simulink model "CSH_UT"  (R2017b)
settings: Solver=FixedStepDiscrete  StartTime=0.0  StopTime=10.0  FixedStep=0.01  RelTol=1e-3  EnableMultiTasking=on
undefined symbols (not defined in the file): ASWTYPE_FALSE, CbCSH_CANCrashFltDetEnable_flg, CcCSH_CshDutyNormalHi_pct, CcCSH_CshDutyNormalLo_pct, CcCSH_CshFltDutyHiThrd_pct, CcCSH_CshFltDutyLoThrd_pct, CcCSH_CshFrqNormalHi_ms, CcCSH_CshFrqNormalLo_ms, CcCSH_DutyAbnormalDetEnable_flg, CcCSH_FrqAbnormalDetEnable_flg, CcCSH_HWCshFltDetEnable_flg, CcCSH_Kl15WkUpDelay_ms, CSH_CONST10_NUMB, CSH_CONST11_NUMB, CSH_CONST16_NUMB, CSH_CONST17_NUMB, CSH_CONST18_NUMB, CSH_CONST19_NUMB, CSH_CONST1_NUMB, CSH_CONST24_NUMB, CSH_CONST25_NUMB, CSH_CONST26_NUMB, CSH_CONST27_NUMB, CSH_CONST2_NUMB, CSH_CONST3_NUMB, CSH_CONST4_NUMB, CSH_CONST5_NUMB, CSH_CONST6_NUMB, CSH_CONST7_NUMB, CSH_CONST8_NUMB, CSH_CONST9_NUMB, CSH_RUNTIME_MS
libraries: AIWAYS_Powertrain_BMS_lib x11

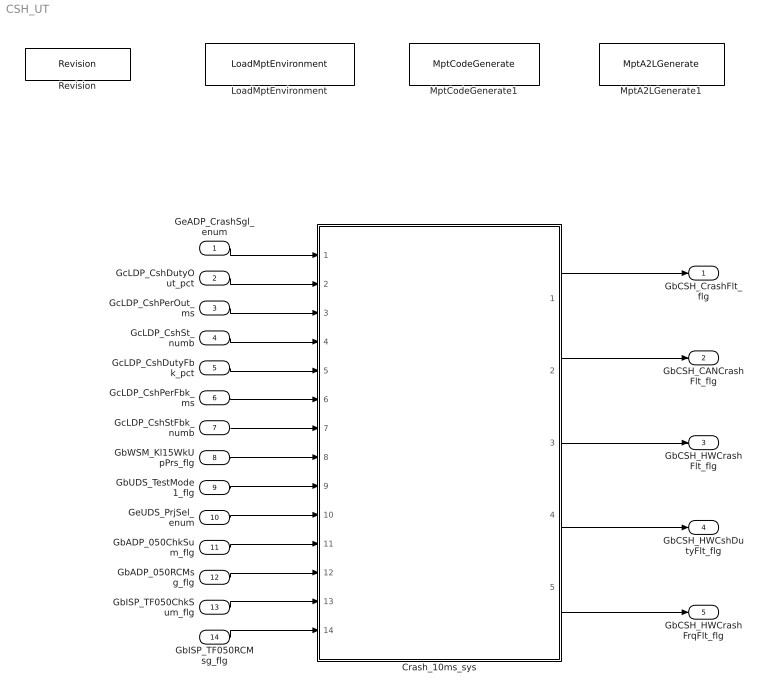
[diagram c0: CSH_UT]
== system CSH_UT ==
  GeADP_CrashSgl_enum : Inport
  GcLDP_CshDutyOut_pct : Inport  Port=2
  GcLDP_CshPerOut_ms : Inport  Port=3
  GcLDP_CshSt_numb : Inport  Port=4
  GcLDP_CshDutyFbk_pct : Inport  Port=5
  GcLDP_CshPerFbk_ms : Inport  Port=6
  GcLDP_CshStFbk_numb : Inport  Port=7
  GbWSM_Kl15WkUpPrs_flg : Inport  Port=8
  GbUDS_TestMode1_flg : Inport  Port=9
  GeUDS_PrjSel_enum : Inport  Port=10
  GbADP_050ChkSum_flg : Inport  Port=11
  GbADP_050RCMsg_flg : Inport  Port=12
  GbISP_TF050ChkSum_flg : Inport  Port=13
  GbISP_TF050RCMsg_flg : Inport  Port=14
  Crash_10ms_sys : Subsystem
  LoadMptEnvironment : AIWAYS_Powertrain_BMS_lib/Config/LoadMptEnvironment  ProjectName=Comm  SuppierID=NewPlatformUAES
  MptA2LGenerate1 : AIWAYS_Powertrain_BMS_lib/Config/MptA2LGenerate  SystemSampleTime=-1
  MptCodeGenerate1 : AIWAYS_Powertrain_BMS_lib/Config/MptCodeGenerate  SystemSampleTime=-1
  Revision : AIWAYS_Powertrain_BMS_lib/Config/Revision  curVersion='M102C102'  newVersion='M102C102'
  GbCSH_CrashFlt_flg : Outport
  GbCSH_CANCrashFlt_flg : Outport  Port=2
  GbCSH_HWCrashFlt_flg : Outport  Port=3
  GbCSH_HWCshDutyFlt_flg : Outport  Port=4
  GbCSH_HWCrashFrqFlt_flg : Outport  Port=5
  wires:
  GcLDP_CshPerOut_ms/1 -> Crash_10ms_sys/3(GcLDP_CshPerOut_ms)
  GcLDP_CshStFbk_numb/1 -> Crash_10ms_sys/7(GcLDP_CshStFbk_numb)
  GbWSM_Kl15WkUpPrs_flg/1 -> Crash_10ms_sys/8(GbWSM_Kl15WkUpPrs_flg)
  Crash_10ms_sys/5(GbCSH_HWCrashFrqFlt_flg) -> GbCSH_HWCrashFrqFlt_flg/1
  GcLDP_CshPerFbk_ms/1 -> Crash_10ms_sys/6(GcLDP_CshPerFbk_ms)
  Crash_10ms_sys/3(GbCSH_HWCrashFlt_flg) -> GbCSH_HWCrashFlt_flg/1
  GbUDS_TestMode1_flg/1 -> Crash_10ms_sys/9(GbUDS_TestMode1_flg)
  Crash_10ms_sys/1(GbCSH_CrashFlt_flg) -> GbCSH_CrashFlt_flg/1
  GeADP_CrashSgl_enum/1 -> Crash_10ms_sys/1(GeADP_CrashSgl_enum)
  GcLDP_CshDutyFbk_pct/1 -> Crash_10ms_sys/5(GcLDP_CshDutyFbk_pct)
  GeUDS_PrjSel_enum/1 -> Crash_10ms_sys/10(GeUDS_PrjSel_enum)
  Crash_10ms_sys/2(GbCSH_CANCrashFlt_flg) -> GbCSH_CANCrashFlt_flg/1
  GbISP_TF050RCMsg_flg/1 -> Crash_10ms_sys/14(GbISP_TF050RCMsg_flg)
  GcLDP_CshSt_numb/1 -> Crash_10ms_sys/4(GcLDP_CshSt_numb)
  GbADP_050ChkSum_flg/1 -> Crash_10ms_sys/11(GbADP_050ChkSum_flg)
  GcLDP_CshDutyOut_pct/1 -> Crash_10ms_sys/2(GcLDP_CshDutyOut_pct)
  Crash_10ms_sys/4(GbCSH_HWCshDutyFlt_flg) -> GbCSH_HWCshDutyFlt_flg/1
  GbADP_050RCMsg_flg/1 -> Crash_10ms_sys/12(GbADP_050RCMsg_flg)
  GbISP_TF050ChkSum_flg/1 -> Crash_10ms_sys/13(GbISP_TF050ChkSum_flg)

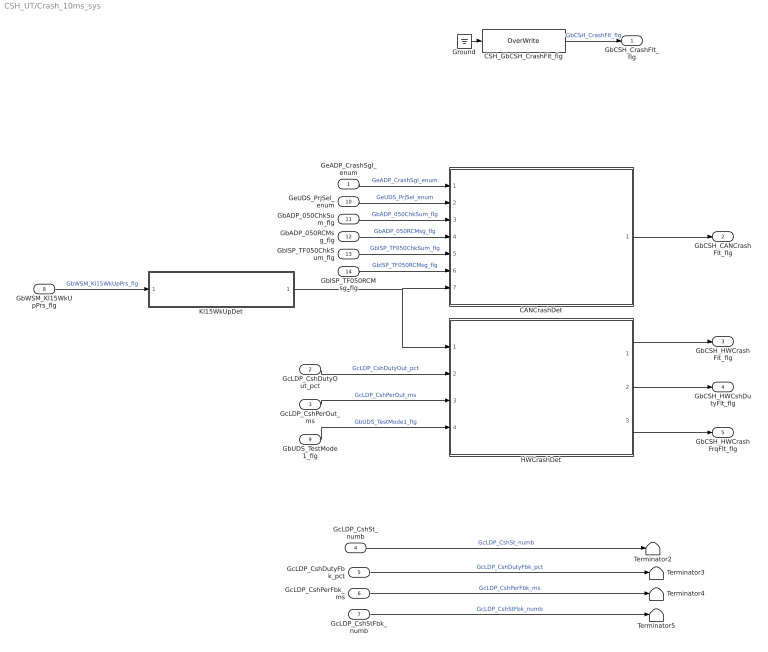
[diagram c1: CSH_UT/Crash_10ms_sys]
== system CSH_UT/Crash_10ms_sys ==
  GeADP_CrashSgl_enum : Inport
  GcLDP_CshDutyOut_pct : Inport  Port=2
  GcLDP_CshPerOut_ms : Inport  Port=3
  GcLDP_CshSt_numb : Inport  Port=4
  GcLDP_CshDutyFbk_pct : Inport  Port=5
  GcLDP_CshPerFbk_ms : Inport  Port=6
  GcLDP_CshStFbk_numb : Inport  Port=7
  GbWSM_Kl15WkUpPrs_flg : Inport  Port=8
  GbUDS_TestMode1_flg : Inport  Port=9
  GeUDS_PrjSel_enum : Inport  Port=10
  GbADP_050ChkSum_flg : Inport  Port=11
  GbADP_050RCMsg_flg : Inport  Port=12
  GbISP_TF050ChkSum_flg : Inport  Port=13
  GbISP_TF050RCMsg_flg : Inport  Port=14
  CANCrashDet : Subsystem
  CSH_GbCSH_CrashFlt_flg : AIWAYS_Powertrain_BMS_lib/Signals/OverWrite  OverWrite_Value=CbCSH_CrashFltOvr_flg  OverWrite_flag=CbCSH_CrashFltOvrSwt_flg
  Ground : Ground
  HWCrashDet : Subsystem
  Kl15WkUpDet : Subsystem
  Terminator{2..5} (4 alike) : Terminator
  GbCSH_CrashFlt_flg : Outport
  GbCSH_CANCrashFlt_flg : Outport  Port=2
  GbCSH_HWCrashFlt_flg : Outport  Port=3
  GbCSH_HWCshDutyFlt_flg : Outport  Port=4
  GbCSH_HWCrashFrqFlt_flg : Outport  Port=5
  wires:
  GeADP_CrashSgl_enum/1 -> CANCrashDet/1(GeADP_CrashSgl_enum)  "GeADP_CrashSgl_enum"
  CSH_GbCSH_CrashFlt_flg/1 -> GbCSH_CrashFlt_flg/1  "GbCSH_CrashFlt_flg"
  GcLDP_CshDutyOut_pct/1 -> HWCrashDet/2(GcLDP_CshDutyOut_pct)  "GcLDP_CshDutyOut_pct"
  GcLDP_CshPerOut_ms/1 -> HWCrashDet/3(GcLDP_CshPerOut_ms)  "GcLDP_CshPerOut_ms"
  GcLDP_CshSt_numb/1 -> Terminator2/1  "GcLDP_CshSt_numb"
  GcLDP_CshDutyFbk_pct/1 -> Terminator3/1  "GcLDP_CshDutyFbk_pct"
  GcLDP_CshPerFbk_ms/1 -> Terminator4/1  "GcLDP_CshPerFbk_ms"
  GcLDP_CshStFbk_numb/1 -> Terminator5/1  "GcLDP_CshStFbk_numb"
  Ground/1 -> CSH_GbCSH_CrashFlt_flg/1
  GbWSM_Kl15WkUpPrs_flg/1 -> Kl15WkUpDet/1(GbWSM_Kl15WkUpPrs_flg)  "GbWSM_Kl15WkUpPrs_flg"
  Kl15WkUpDet/1(LbCSH_Kl15WkUpPrs_flg) -> HWCrashDet/1(LbCSH_Kl15WkUpPrs_flg), CANCrashDet/7(LbCSH_Kl15WkUpPrs_flg)
  GbUDS_TestMode1_flg/1 -> HWCrashDet/4(GbUDS_TestMode1_flg)  "GbUDS_TestMode1_flg"
  GeUDS_PrjSel_enum/1 -> CANCrashDet/2(GeUDS_PrjSel_enum)  "GeUDS_PrjSel_enum"
  HWCrashDet/1(GbCSH_HWCrashFlt_flg) -> GbCSH_HWCrashFlt_flg/1
  HWCrashDet/2(GbCSH_HWCshDutyFlt_flg) -> GbCSH_HWCshDutyFlt_flg/1
  HWCrashDet/3(GbCSH_HWCrashFrqFlt_flg) -> GbCSH_HWCrashFrqFlt_flg/1
  GbADP_050ChkSum_flg/1 -> CANCrashDet/3(GbADP_050ChkSum_flg)  "GbADP_050ChkSum_flg"
  GbADP_050RCMsg_flg/1 -> CANCrashDet/4(GbADP_050RCMsg_flg)  "GbADP_050RCMsg_flg"
  GbISP_TF050ChkSum_flg/1 -> CANCrashDet/5(GbISP_TF050ChkSum_flg)  "GbISP_TF050ChkSum_flg"
  GbISP_TF050RCMsg_flg/1 -> CANCrashDet/6(GbISP_TF050RCMsg_flg)  "GbISP_TF050RCMsg_flg"
  CANCrashDet/1(GbCSH_CANCrashFlt_flg) -> GbCSH_CANCrashFlt_flg/1

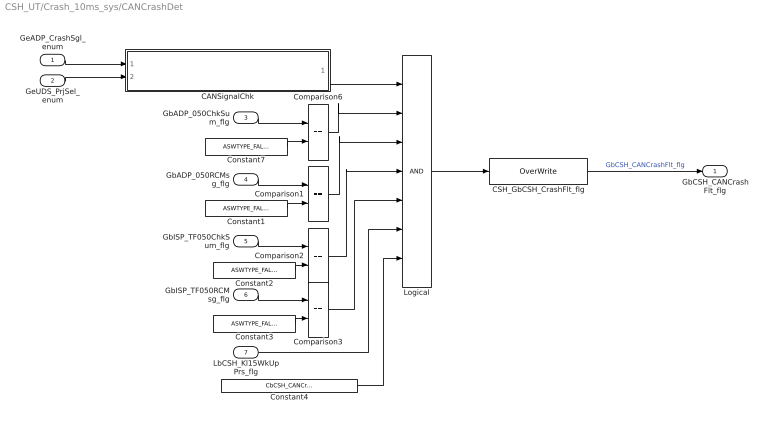
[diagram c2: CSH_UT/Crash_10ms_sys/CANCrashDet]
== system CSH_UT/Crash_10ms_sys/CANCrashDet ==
  GeADP_CrashSgl_enum : Inport
  GeUDS_PrjSel_enum : Inport  Port=2
  GbADP_050ChkSum_flg : Inport  Port=3
  GbADP_050RCMsg_flg : Inport  Port=4
  GbISP_TF050ChkSum_flg : Inport  Port=5
  GbISP_TF050RCMsg_flg : Inport  Port=6
  LbCSH_Kl15WkUpPrs_flg : Inport  Port=7
  CANSignalChk : Subsystem
  CSH_GbCSH_CrashFlt_flg : AIWAYS_Powertrain_BMS_lib/Signals/OverWrite  OverWrite_Value=CbCSH_CANCrashFltOvr_flg  OverWrite_flag=CbCSH_CANCrashFltOvrSwt_flg
  Comparison{1..3,6} (4 alike) : RelationalOperator  Operator===  OutDataTypeStr=boolean
  Constant{1..3,7} (4 alike) : Constant  Value=ASWTYPE_FALSE
  Constant4 : Constant  Value=CbCSH_CANCrashFltDetEnable_flg
  Logical : Logic  Inputs=7  OutDataTypeStr=boolean
  GbCSH_CANCrashFlt_flg : Outport
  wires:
  LbCSH_Kl15WkUpPrs_flg/1 -> Logical/6
  GeADP_CrashSgl_enum/1 -> CANSignalChk/1(GeADP_CrashSgl_enum)
  GeUDS_PrjSel_enum/1 -> CANSignalChk/2(GeUDS_PrjSel_enum)
  Constant7/1 -> Comparison6/2
  GbADP_050ChkSum_flg/1 -> Comparison6/1
  Constant1/1 -> Comparison1/2
  GbADP_050RCMsg_flg/1 -> Comparison1/1
  CANSignalChk/1(LbCSH_CANCrashState_flg) -> Logical/1
  Comparison6/1 -> Logical/2
  Comparison1/1 -> Logical/3
  GbISP_TF050ChkSum_flg/1 -> Comparison2/1
  Constant2/1 -> Comparison2/2
  Comparison2/1 -> Logical/4
  GbISP_TF050RCMsg_flg/1 -> Comparison3/1
  Constant3/1 -> Comparison3/2
  Comparison3/1 -> Logical/5
  Logical/1 -> CSH_GbCSH_CrashFlt_flg/1
  CSH_GbCSH_CrashFlt_flg/1 -> GbCSH_CANCrashFlt_flg/1  "GbCSH_CANCrashFlt_flg"
  Constant4/1 -> Logical/7

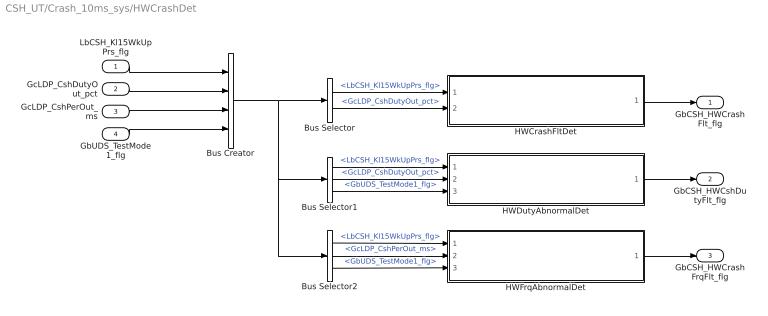
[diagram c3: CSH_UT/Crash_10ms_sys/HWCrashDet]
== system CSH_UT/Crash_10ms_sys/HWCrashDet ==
  LbCSH_Kl15WkUpPrs_flg : Inport
  GcLDP_CshDutyOut_pct : Inport  Port=2
  GcLDP_CshPerOut_ms : Inport  Port=3
  GbUDS_TestMode1_flg : Inport  Port=4
  Bus Creator : BusCreator  Inputs=4
  Bus Selector : BusSelector  OutputSignals=LbCSH_Kl15WkUpPrs_flg,GcLDP_CshDutyOut_pct
  Bus Selector1 : BusSelector  OutputSignals=LbCSH_Kl15WkUpPrs_flg,GcLDP_CshDutyOut_pct,GbUDS_TestMode1_flg
  Bus Selector2 : BusSelector  OutputSignals=LbCSH_Kl15WkUpPrs_flg,GcLDP_CshPerOut_ms,GbUDS_TestMode1_flg
  HWCrashFltDet : Subsystem
  HWDutyAbnormalDet : Subsystem
  HWFrqAbnormalDet : Subsystem
  GbCSH_HWCrashFlt_flg : Outport
  GbCSH_HWCshDutyFlt_flg : Outport  Port=2
  GbCSH_HWCrashFrqFlt_flg : Outport  Port=3
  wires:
  LbCSH_Kl15WkUpPrs_flg/1 -> Bus Creator/1
  GcLDP_CshDutyOut_pct/1 -> Bus Creator/2
  GcLDP_CshPerOut_ms/1 -> Bus Creator/3
  Bus Creator/1 -> Bus Selector2/1, Bus Selector1/1, Bus Selector/1
  Bus Selector/1 -> HWCrashFltDet/1(LbCSH_Kl15WkUpPrs_flg)  "<LbCSH_Kl15WkUpPrs_flg>"
  Bus Selector/2 -> HWCrashFltDet/2(GcLDP_CshDutyOut_pct)  "<GcLDP_CshDutyOut_pct>"
  GbUDS_TestMode1_flg/1 -> Bus Creator/4
  HWCrashFltDet/1(GbCSH_HWCrashFlt_flg) -> GbCSH_HWCrashFlt_flg/1
  Bus Selector1/1 -> HWDutyAbnormalDet/1(LbCSH_Kl15WkUpPrs_flg)  "<LbCSH_Kl15WkUpPrs_flg>"
  Bus Selector1/2 -> HWDutyAbnormalDet/2(GcLDP_CshDutyOut_pct)  "<GcLDP_CshDutyOut_pct>"
  Bus Selector1/3 -> HWDutyAbnormalDet/3(GbUDS_TestMode1_flg)  "<GbUDS_TestMode1_flg>"
  Bus Selector2/1 -> HWFrqAbnormalDet/1(LbCSH_Kl15WkUpPrs_flg)  "<LbCSH_Kl15WkUpPrs_flg>"
  Bus Selector2/2 -> HWFrqAbnormalDet/2(GcLDP_CshPerOut_ms)  "<GcLDP_CshPerOut_ms>"
  Bus Selector2/3 -> HWFrqAbnormalDet/3(GbUDS_TestMode1_flg)  "<GbUDS_TestMode1_flg>"
  HWDutyAbnormalDet/1(GbCSH_HWCshDutyFlt_flg) -> GbCSH_HWCshDutyFlt_flg/1
  HWFrqAbnormalDet/1(GbCSH_HWCrashFrqFlt_flg) -> GbCSH_HWCrashFrqFlt_flg/1

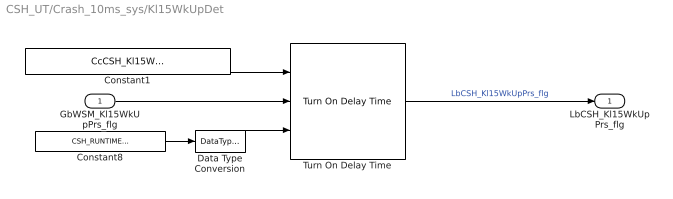
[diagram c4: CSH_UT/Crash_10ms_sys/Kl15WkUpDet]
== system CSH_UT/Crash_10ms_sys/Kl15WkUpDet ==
  GbWSM_Kl15WkUpPrs_flg : Inport
  Constant1 : Constant  Value=CcCSH_Kl15WkUpDelay_ms
  Constant8 : Constant  Value=CSH_RUNTIME_MS
  Data Type Conversion : DataTypeConversion
  Turn On Delay Time : AIWAYS_Powertrain_BMS_lib/Delay Blocks/Turn On Delay Time
  LbCSH_Kl15WkUpPrs_flg : Outport
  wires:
  GbWSM_Kl15WkUpPrs_flg/1 -> Turn On Delay Time/2
  Constant8/1 -> Data Type Conversion/1
  Constant1/1 -> Turn On Delay Time/1
  Turn On Delay Time/1 -> LbCSH_Kl15WkUpPrs_flg/1  "LbCSH_Kl15WkUpPrs_flg"
  Data Type Conversion/1 -> Turn On Delay Time/3

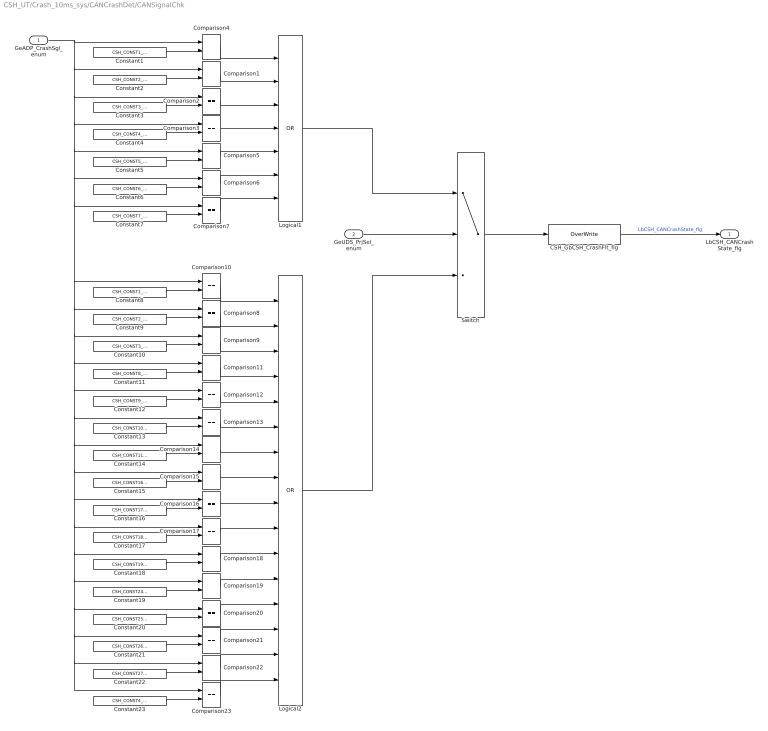
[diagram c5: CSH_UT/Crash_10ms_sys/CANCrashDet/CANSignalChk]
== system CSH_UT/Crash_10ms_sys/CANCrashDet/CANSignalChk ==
  GeADP_CrashSgl_enum : Inport
  GeUDS_PrjSel_enum : Inport  Port=2
  CSH_GbCSH_CrashFlt_flg : AIWAYS_Powertrain_BMS_lib/Signals/OverWrite  OverWrite_Value=CbCSH_CANCrashStateOvr_flg  OverWrite_flag=CbCSH_CANCrashStateOvrSwt_flg
  Comparison{1..23} (23 alike) : RelationalOperator  Operator===  OutDataTypeStr=boolean
  Constant1 : Constant  Value=CSH_CONST1_NUMB
  Constant10 : Constant  Value=CSH_CONST3_NUMB
  Constant11 : Constant  Value=CSH_CONST8_NUMB
  Constant12 : Constant  Value=CSH_CONST9_NUMB
  Constant13 : Constant  Value=CSH_CONST10_NUMB
  Constant14 : Constant  Value=CSH_CONST11_NUMB
  Constant15 : Constant  Value=CSH_CONST16_NUMB
  Constant16 : Constant  Value=CSH_CONST17_NUMB
  Constant17 : Constant  Value=CSH_CONST18_NUMB
  Constant18 : Constant  Value=CSH_CONST19_NUMB
  Constant19 : Constant  Value=CSH_CONST24_NUMB
  Constant2 : Constant  Value=CSH_CONST2_NUMB
  Constant20 : Constant  Value=CSH_CONST25_NUMB
  Constant21 : Constant  Value=CSH_CONST26_NUMB
  Constant22 : Constant  Value=CSH_CONST27_NUMB
  Constant23 : Constant  Value=CSH_CONST4_NUMB
  Constant3 : Constant  Value=CSH_CONST3_NUMB
  Constant4 : Constant  Value=CSH_CONST4_NUMB
  Constant5 : Constant  Value=CSH_CONST5_NUMB
  Constant6 : Constant  Value=CSH_CONST6_NUMB
  Constant7 : Constant  Value=CSH_CONST7_NUMB
  Constant8 : Constant  Value=CSH_CONST1_NUMB
  Constant9 : Constant  Value=CSH_CONST2_NUMB
  Logical1 : Logic  Operator=OR  Inputs=7  OutDataTypeStr=boolean
  Logical2 : Logic  Operator=OR  Inputs=16  OutDataTypeStr=boolean
  Switch : Switch  Criteria=u2 ~= 0  Threshold=1  RndMeth=Zero
  LbCSH_CANCrashState_flg : Outport
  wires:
  Constant1/1 -> Comparison4/2
  Constant2/1 -> Comparison1/2
  Constant3/1 -> Comparison2/2
  Constant4/1 -> Comparison3/2
  Constant5/1 -> Comparison5/2
  Constant6/1 -> Comparison6/2
  Constant7/1 -> Comparison7/2
  Comparison4/1 -> Logical1/1
  Comparison1/1 -> Logical1/2
  Comparison2/1 -> Logical1/3
  Comparison3/1 -> Logical1/4
  Comparison5/1 -> Logical1/5
  Comparison6/1 -> Logical1/6
  Comparison7/1 -> Logical1/7
  GeADP_CrashSgl_enum/1 -> Comparison2/1, Comparison3/1, Comparison5/1, Comparison6/1, Comparison7/1, Comparison9/1, Comparison14/1, Comparison15/1, Comparison16/1, Comparison17/1, Comparison18/1, Comparison19/1, Comparison20/1, Comparison21/1, Comparison23/1, Comparison22/1, Comparison13/1, Comparison12/1, Comparison11/1, Comparison8/1, Comparison10/1, Comparison1/1, Comparison4/1
  Constant9/1 -> Comparison8/2
  Constant8/1 -> Comparison10/2
  Constant10/1 -> Comparison9/2
  Constant11/1 -> Comparison11/2
  Constant12/1 -> Comparison12/2
  Constant13/1 -> Comparison13/2
  Constant14/1 -> Comparison14/2
  Constant18/1 -> Comparison18/2
  Constant17/1 -> Comparison17/2
  Constant16/1 -> Comparison16/2
  Constant15/1 -> Comparison15/2
  Constant19/1 -> Comparison19/2
  Constant20/1 -> Comparison20/2
  Constant21/1 -> Comparison21/2
  Constant22/1 -> Comparison22/2
  Comparison10/1 -> Logical2/1
  Comparison8/1 -> Logical2/2
  Comparison9/1 -> Logical2/3
  Comparison11/1 -> Logical2/4
  Comparison12/1 -> Logical2/5
  Comparison13/1 -> Logical2/6
  Comparison14/1 -> Logical2/7
  Comparison15/1 -> Logical2/8
  Comparison16/1 -> Logical2/9
  Comparison17/1 -> Logical2/10
  Comparison18/1 -> Logical2/11
  Comparison19/1 -> Logical2/12
  Comparison20/1 -> Logical2/13
  Comparison21/1 -> Logical2/14
  Comparison22/1 -> Logical2/15
  Logical1/1 -> Switch/1
  GeUDS_PrjSel_enum/1 -> Switch/2
  Logical2/1 -> Switch/3
  Switch/1 -> CSH_GbCSH_CrashFlt_flg/1
  CSH_GbCSH_CrashFlt_flg/1 -> LbCSH_CANCrashState_flg/1  "LbCSH_CANCrashState_flg"
  Constant23/1 -> Comparison23/2
  Comparison23/1 -> Logical2/16

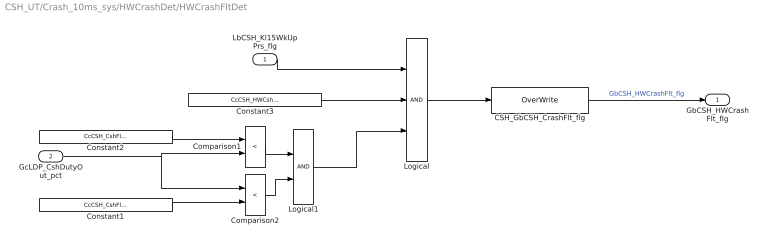
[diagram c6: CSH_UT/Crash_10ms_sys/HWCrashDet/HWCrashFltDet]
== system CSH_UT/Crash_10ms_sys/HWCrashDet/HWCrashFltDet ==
  LbCSH_Kl15WkUpPrs_flg : Inport
  GcLDP_CshDutyOut_pct : Inport  Port=2
  CSH_GbCSH_CrashFlt_flg : AIWAYS_Powertrain_BMS_lib/Signals/OverWrite  OverWrite_Value=CbCSH_HWCrashFltOvr_flg  OverWrite_flag=CbCSH_HWCrashFltOvrSwt_flg
  Comparison1 : RelationalOperator  Operator=<  OutDataTypeStr=boolean
  Comparison2 : RelationalOperator  Operator=<  OutDataTypeStr=boolean
  Constant1 : Constant  Value=CcCSH_CshFltDutyHiThrd_pct
  Constant2 : Constant  Value=CcCSH_CshFltDutyLoThrd_pct
  Constant3 : Constant  Value=CcCSH_HWCshFltDetEnable_flg
  Logical : Logic  Inputs=3  OutDataTypeStr=boolean
  Logical1 : Logic  OutDataTypeStr=boolean
  GbCSH_HWCrashFlt_flg : Outport
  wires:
  Constant1/1 -> Comparison2/2
  GcLDP_CshDutyOut_pct/1 -> Comparison2/1, Comparison1/2
  Constant2/1 -> Comparison1/1
  Comparison1/1 -> Logical1/1
  Comparison2/1 -> Logical1/2
  LbCSH_Kl15WkUpPrs_flg/1 -> Logical/1
  Constant3/1 -> Logical/2
  Logical1/1 -> Logical/3
  Logical/1 -> CSH_GbCSH_CrashFlt_flg/1
  CSH_GbCSH_CrashFlt_flg/1 -> GbCSH_HWCrashFlt_flg/1  "GbCSH_HWCrashFlt_flg"

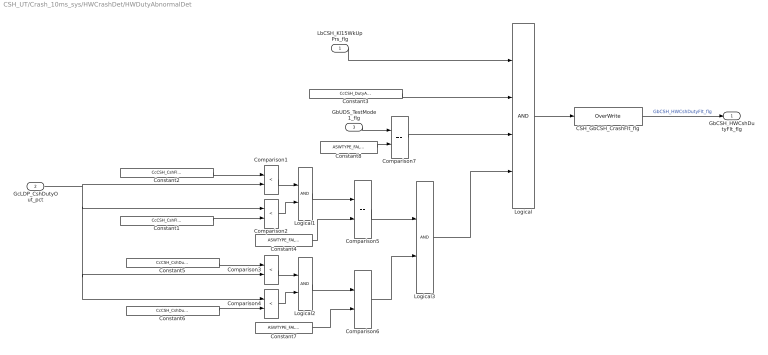
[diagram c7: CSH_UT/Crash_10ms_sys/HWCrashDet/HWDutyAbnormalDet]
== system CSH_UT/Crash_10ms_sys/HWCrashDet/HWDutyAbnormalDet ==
  LbCSH_Kl15WkUpPrs_flg : Inport
  GcLDP_CshDutyOut_pct : Inport  Port=2
  GbUDS_TestMode1_flg : Inport  Port=3
  CSH_GbCSH_CrashFlt_flg : AIWAYS_Powertrain_BMS_lib/Signals/OverWrite  OverWrite_Value=CbCSH_HWCshDutyFltOvr_flg  OverWrite_flag=CbCSH_HWCshDutyFltOvrSwt_flg
  Comparison{1..4} (4 alike) : RelationalOperator  Operator=<  OutDataTypeStr=boolean
  Comparison5 : RelationalOperator  Operator===  OutDataTypeStr=boolean
  Comparison6 : RelationalOperator  Operator===  OutDataTypeStr=boolean
  Comparison7 : RelationalOperator  Operator===  OutDataTypeStr=boolean
  Constant1 : Constant  Value=CcCSH_CshFltDutyHiThrd_pct
  Constant2 : Constant  Value=CcCSH_CshFltDutyLoThrd_pct
  Constant3 : Constant  Value=CcCSH_DutyAbnormalDetEnable_flg
  Constant4 : Constant  Value=ASWTYPE_FALSE
  Constant5 : Constant  Value=CcCSH_CshDutyNormalLo_pct
  Constant6 : Constant  Value=CcCSH_CshDutyNormalHi_pct
  Constant7 : Constant  Value=ASWTYPE_FALSE
  Constant8 : Constant  Value=ASWTYPE_FALSE
  Logical : Logic  Inputs=4  OutDataTypeStr=boolean
  Logical1 : Logic  OutDataTypeStr=boolean
  Logical2 : Logic  OutDataTypeStr=boolean
  Logical3 : Logic  OutDataTypeStr=boolean
  GbCSH_HWCshDutyFlt_flg : Outport
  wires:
  CSH_GbCSH_CrashFlt_flg/1 -> GbCSH_HWCshDutyFlt_flg/1  "GbCSH_HWCshDutyFlt_flg"
  Logical/1 -> CSH_GbCSH_CrashFlt_flg/1
  Logical1/1 -> Comparison5/1
  Constant3/1 -> Logical/2
  LbCSH_Kl15WkUpPrs_flg/1 -> Logical/1
  Comparison2/1 -> Logical1/2
  Comparison1/1 -> Logical1/1
  Constant2/1 -> Comparison1/1
  Constant1/1 -> Comparison2/2
  Constant5/1 -> Comparison3/1
  GcLDP_CshDutyOut_pct/1 -> Comparison1/2, Comparison3/2, Comparison4/1, Comparison2/1
  Constant6/1 -> Comparison4/2
  Comparison3/1 -> Logical2/1
  Comparison4/1 -> Logical2/2
  Constant4/1 -> Comparison5/2
  Logical2/1 -> Comparison6/1
  Constant7/1 -> Comparison6/2
  GbUDS_TestMode1_flg/1 -> Comparison7/1
  Constant8/1 -> Comparison7/2
  Comparison5/1 -> Logical3/1
  Comparison6/1 -> Logical3/2
  Comparison7/1 -> Logical/3
  Logical3/1 -> Logical/4

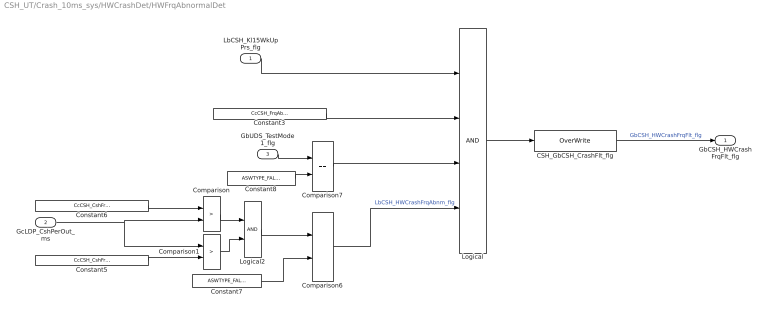
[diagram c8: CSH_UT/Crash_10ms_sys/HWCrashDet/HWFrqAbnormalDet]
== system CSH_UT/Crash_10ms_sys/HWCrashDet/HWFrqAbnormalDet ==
  LbCSH_Kl15WkUpPrs_flg : Inport
  GcLDP_CshPerOut_ms : Inport  Port=2
  GbUDS_TestMode1_flg : Inport  Port=3
  CSH_GbCSH_CrashFlt_flg : AIWAYS_Powertrain_BMS_lib/Signals/OverWrite  OverWrite_Value=CbCSH_HWCrashFrqFltOvr_flg  OverWrite_flag=CbCSH_HWCrashFrqFltOvrSwt_flg
  Comparison : RelationalOperator  Operator=>  OutDataTypeStr=boolean
  Comparison1 : RelationalOperator  Operator=>  OutDataTypeStr=boolean
  Comparison6 : RelationalOperator  Operator===  OutDataTypeStr=boolean
  Comparison7 : RelationalOperator  Operator===  OutDataTypeStr=boolean
  Constant3 : Constant  Value=CcCSH_FrqAbnormalDetEnable_flg
  Constant5 : Constant  Value=CcCSH_CshFrqNormalLo_ms
  Constant6 : Constant  Value=CcCSH_CshFrqNormalHi_ms
  Constant7 : Constant  Value=ASWTYPE_FALSE
  Constant8 : Constant  Value=ASWTYPE_FALSE
  Logical : Logic  Inputs=4  OutDataTypeStr=boolean
  Logical2 : Logic  OutDataTypeStr=boolean
  GbCSH_HWCrashFrqFlt_flg : Outport
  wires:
  Comparison6/1 -> Logical/4  "LbCSH_HWCrashFrqAbnm_flg"
  Comparison7/1 -> Logical/3
  Constant8/1 -> Comparison7/2
  GbUDS_TestMode1_flg/1 -> Comparison7/1
  Constant7/1 -> Comparison6/2
  Logical2/1 -> Comparison6/1
  Comparison1/1 -> Logical2/2
  Comparison/1 -> Logical2/1
  Constant6/1 -> Comparison/1
  GcLDP_CshPerOut_ms/1 -> Comparison1/1, Comparison/2
  Constant5/1 -> Comparison1/2
  LbCSH_Kl15WkUpPrs_flg/1 -> Logical/1
  Constant3/1 -> Logical/2
  Logical/1 -> CSH_GbCSH_CrashFlt_flg/1
  CSH_GbCSH_CrashFlt_flg/1 -> GbCSH_HWCrashFrqFlt_flg/1  "GbCSH_HWCrashFrqFlt_flg"
